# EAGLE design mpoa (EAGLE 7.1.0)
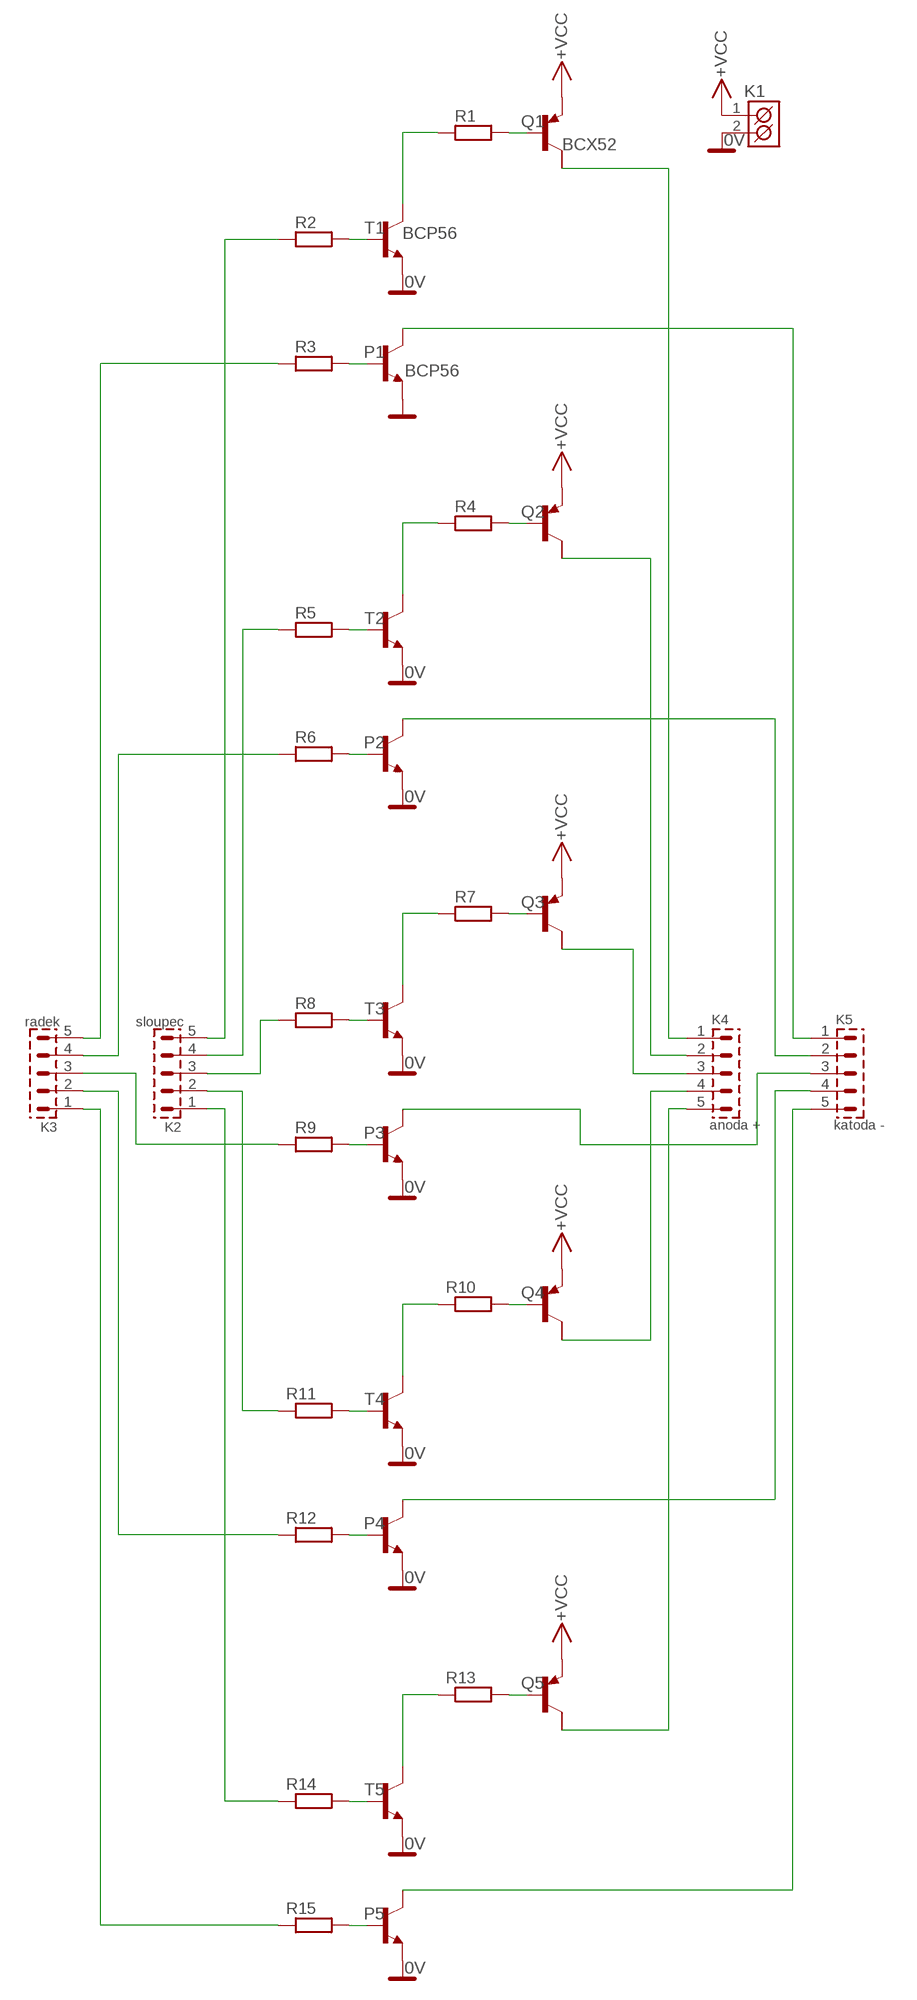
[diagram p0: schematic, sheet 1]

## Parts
K1  ARK550/2  [ARK550/2]
K2  sloupec  PSH02-05P  [PSH02-05P]
K3  radek  PSH02-05P  [PSH02-05P]
K4  anoda +  PSH02-05P  [PSH02-05P]
K5  katoda -  PSH02-05P  [PSH02-05P]
P1  -NPN-SOT223  [SOT223]
P2  -NPN-SOT223  [SOT223]
P3  -NPN-SOT223  [SOT223]
P4  -NPN-SOT223  [SOT223]
P5  -NPN-SOT223  [SOT223]
Q1  BCX52  PNP-TRANSISTIOR-2COLSOT89  [SOT89]
Q2  PNP-TRANSISTIOR-2COLSOT89  [SOT89]
Q3  PNP-TRANSISTIOR-2COLSOT89  [SOT89]
Q4  PNP-TRANSISTIOR-2COLSOT89  [SOT89]
Q5  PNP-TRANSISTIOR-2COLSOT89  [SOT89]
R1  R_1206  [1206]
R2  R_1206  [1206]
R3  R_1206  [1206]
R4  R_1206  [1206]
R5  R_1206  [1206]
R6  R_1206  [1206]
R7  R_1206  [1206]
R8  R_1206  [1206]
R9  R_1206  [1206]
R10  R_1206  [1206]
R11  R_1206  [1206]
R12  R_1206  [1206]
R13  R_1206  [1206]
R14  R_1206  [1206]
R15  R_1206  [1206]
T1  BCP56  -NPN-SOT223  [SOT223]
T2  -NPN-SOT223  [SOT223]
T3  -NPN-SOT223  [SOT223]
T4  -NPN-SOT223  [SOT223]
T5  -NPN-SOT223  [SOT223]

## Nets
0V: K1.2(K2) P1.3(E) P2.3(E) P3.3(E) P4.3(E) P5.3(E) T1.3(E) T2.3(E) T3.3(E) T4.3(E) T5.3(E) ; supply symbol labelled BCP56
N$1: K2.5 R2.1
N$2: R1.1 T1.4(C)
N$3: R2.2 T1.1(B)
N$4: Q1.1(B) R1.2
N$5: P1.1(B) R3.2
N$6: K2.3 R8.1
N$8: K4.1 Q1.2(C)
N$9: R5.2 T2.1(B)
N$10: Q2.1(B) R4.2
N$11: R4.1 T2.4(C)
N$12: P2.1(B) R6.2
N$13: K5.2 P2.4(C)
N$14: K4.2 Q2.2(C)
N$15: R8.2 T3.1(B)
N$16: Q3.1(B) R7.2
N$17: R7.1 T3.4(C)
N$18: P3.1(B) R9.2
N$19: K5.3 P3.4(C)
N$20: K4.3 Q3.2(C)
N$21: R11.2 T4.1(B)
N$22: Q4.1(B) R10.2
N$23: R10.1 T4.4(C)
N$24: P4.1(B) R12.2
N$25: K5.4 P4.4(C)
N$26: K4.4 Q4.2(C)
N$27: R14.2 T5.1(B)
N$28: Q5.1(B) R13.2
N$29: R13.1 T5.4(C)
N$30: P5.1(B) R15.2
N$32: K4.5 Q5.2(C)
N$34: K3.5 R3.1
N$35: K2.1 R14.1
N$36: K3.1 R15.1
N$37: K2.2 R11.1
N$38: K3.2 R12.1
N$39: K3.4 R6.1
N$40: K2.4 R5.1
N$41: K3.3 R9.1
N$42: K5.1 P1.4(C)
N$44: K5.5 P5.4(C)
VCC: K1.1(K1) Q1.3(E) Q2.3(E) Q3.3(E) Q4.3(E) Q5.3(E) ; supply symbol labelled +VCC
Unconnected: Q1.2@1(C/) Q2.2@1(C/) Q3.2@1(C/) Q4.2@1(C/) Q5.2@1(C/)

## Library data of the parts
K1 = #PaJa_konektory:ARK550/2: Svorkovnice - roztec 3,5mm - dvojita
K2-K5 = #PaJa_konektory:PSH02-05: Konektory se zamkem - vidlice - 5pin
P1-P5 T1-T5 = transistor-neu-to92:*-NPN-: NPN Transistror
Q1-Q5 = semicon-smd-ipc:PNP-TRANSISTIOR-2COL: PNP TRANSISTOR 2 colletor pins
R1-R15 = #PaJa_31:R: Rezistor

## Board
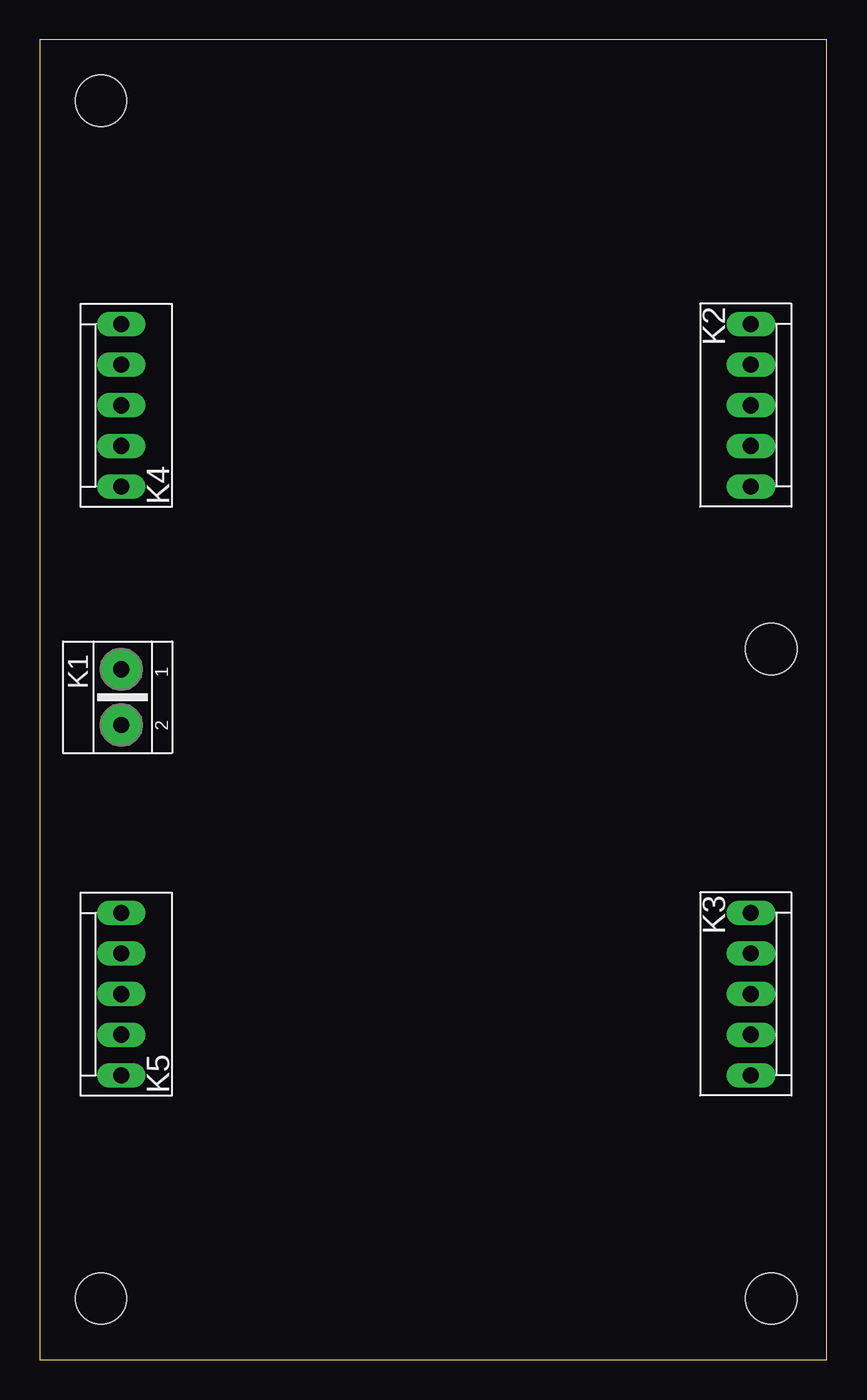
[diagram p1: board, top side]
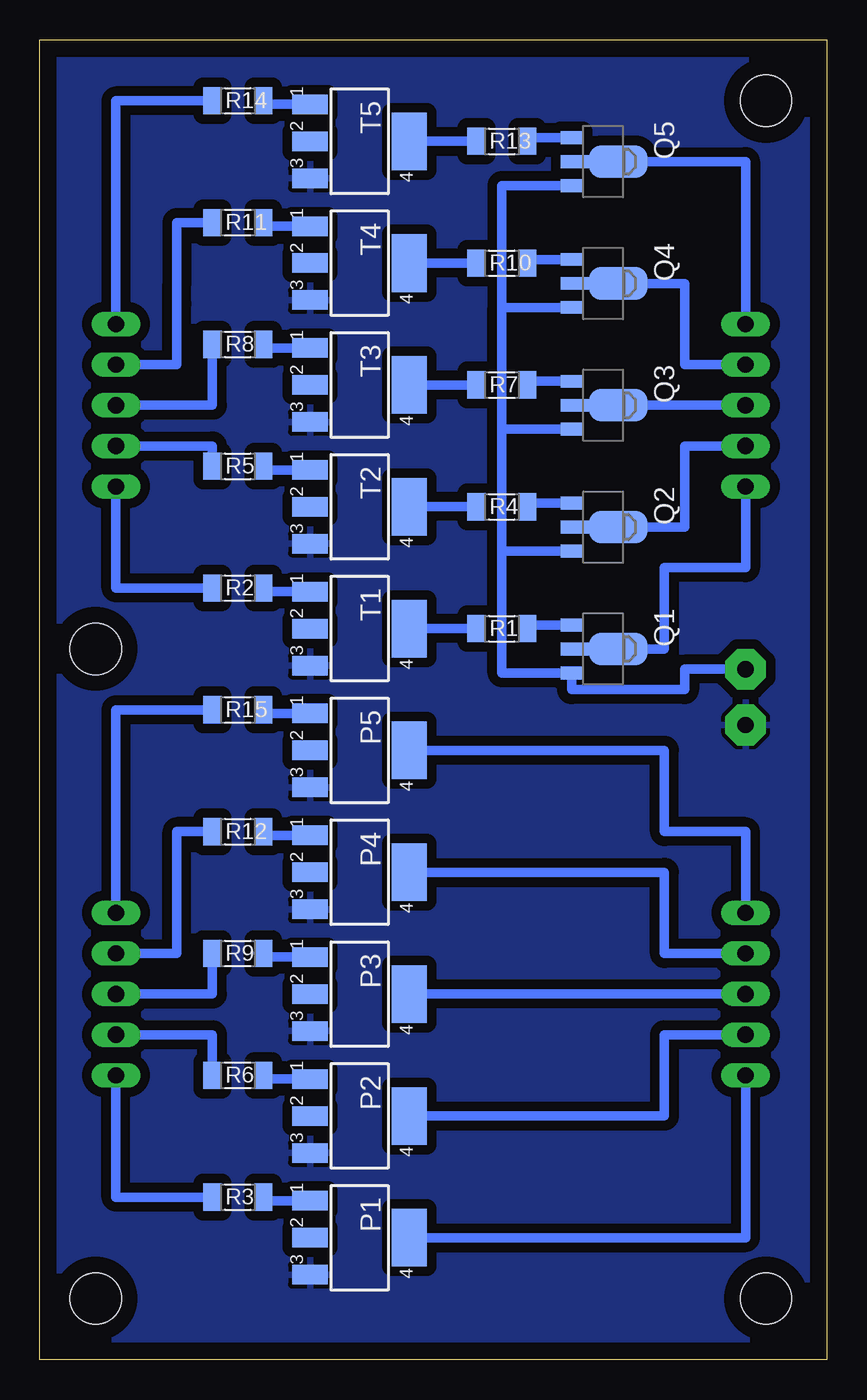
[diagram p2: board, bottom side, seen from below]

Size 49.2 x 82.54 mm. Coordinates in mm from the lower left corner, seen from the top.
Outline: 0,0 49.2,0 49.2,82.54 0,82.54 0,0
Copper layers (1*16): Top 0.035mm / dielectric 1.5mm / Bottom 0.035mm
Design rules "default": minimum track width 10mil, minimum drill 24mil, track to track 8mil, track to pad 8mil, pad to pad 8mil, via to via 8mil, smd to smd 8mil, copper to edge 40mil, drill to drill 8mil, minimum pad ring 10mil, minimum via ring 8mil, stop-mask expansion 4mil, vias tented up to drill 0mil, thermal gap 10mil
Holes 3.2 mm at 3.81,78.74 3.81,3.81 45.72,3.81 45.72,44.45

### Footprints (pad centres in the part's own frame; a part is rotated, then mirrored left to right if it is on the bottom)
ARK550/2 = drill 1.016 pad 2.54 octagon: 1 0,0; 2 3.493,0
PSH02-05P = drill 1.016 pad 1.422 long: 1 -5.08,0; 2 -2.54,0; 3 0,0; 4 2.54,0; 5 5.08,0
SOT223 = smd 1.219 x 2.235: 1 -2.311,-3.099; 2 0,-3.099; 3 2.311,-3.099 | smd 3.6 x 2.2: 4 0,3.099
SOT89 = smd 0.8 x 1.4: 1 -1.499,-1.981; 3 1.499,-1.981 | smd 0.8 x 1.9: 2 0,-1.727 | smd 2.032 x 3.65: 2@1 0,0.94
1206 = smd 1.143 x 1.702: 1 -1.587,0; 2 1.587,0

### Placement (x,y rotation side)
K1  5.08,43.18 270 top
K2  44.45,59.69 270 top
K3  44.45,22.86 270 top
K4  5.08,59.69 90 top
K5  5.08,22.86 90 top
P1  29.21,7.62 270 bottom
P2  29.21,15.24 270 bottom
P3  29.21,22.86 270 bottom
P4  29.21,30.48 270 bottom
P5  29.21,38.1 270 bottom
Q1  13.97,44.45 270 bottom
Q2  13.97,52.07 270 bottom
Q3  13.97,59.69 270 bottom
Q4  13.97,67.31 270 bottom
Q5  13.97,74.93 270 bottom
R1  20.32,45.72 0 bottom
R2  36.83,48.26 0 bottom
R3  36.83,10.16 0 bottom
R4  20.32,53.34 0 bottom
R5  36.83,55.88 0 bottom
R6  36.83,17.78 0 bottom
R7  20.32,60.96 0 bottom
R8  36.83,63.5 0 bottom
R9  36.83,25.4 0 bottom
R10  20.32,68.58 0 bottom
R11  36.83,71.12 0 bottom
R12  36.83,33.02 0 bottom
R13  20.32,76.2 0 bottom
R14  36.83,78.74 0 bottom
R15  36.83,40.64 0 bottom
T1  29.21,45.72 270 bottom
T2  29.21,53.34 270 bottom
T3  29.21,60.96 270 bottom
T4  29.21,68.58 270 bottom
T5  29.21,76.2 270 bottom

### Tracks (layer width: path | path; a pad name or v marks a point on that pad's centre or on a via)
0V
  pour Bottom (isolate 0.61): 1.27,81.28 48.26,81.28 48.26,1.27 1.27,1.27
N$1
  Bottom 0.61: R2.1 44.45,48.26 K2.5
N$2
  Bottom 0.61: R1.1 T1.4
N$3
  Bottom 0.61: T1.1 35.24,48.03 R2.2
N$4
  Bottom 0.61: Q1.1 18.73,45.95 R1.2
N$5
  Bottom 0.61: P1.1 35.24,9.93 R3.2
N$6
  Bottom 0.61: K2.3 38.42,59.69 R8.1
N$8
  Bottom 0.61: Q1.2 10.16,44.45 10.16,49.53 5.08,49.53 K4.1
N$9
  Bottom 0.61: T2.1 35.24,55.65 R5.2
N$10
  Bottom 0.61: Q2.1 18.73,53.57 R4.2
N$11
  Bottom 0.61: R4.1 T2.4
N$12
  Bottom 0.61: P2.1 35.24,17.55 R6.2
N$13
  Bottom 0.61: P2.4 10.16,15.24 10.16,20.32 K5.2
N$14
  Bottom 0.61: Q2.2 8.89,52.07 8.89,57.15 K4.2
N$15
  Bottom 0.61: T3.1 35.24,63.27 R8.2
N$16
  Bottom 0.61: Q3.1 18.73,61.19 R7.2
N$17
  Bottom 0.61: R7.1 T3.4
N$18
  Bottom 0.61: 35.56,25.4 R9.2 35.24,25.17 P3.1
N$19
  Bottom 0.61: K5.3 P3.4
N$20
  Bottom 0.61: K4.3 Q3.2
N$21
  Bottom 0.61: T4.1 35.24,70.89 R11.2
N$22
  Bottom 0.61: Q4.1 18.73,68.81 R10.2
N$23
  Bottom 0.61: R10.1 T4.4
N$24
  Bottom 0.61: P4.1 35.24,32.79 R12.2
N$25
  Bottom 0.61: P4.4 10.16,30.48 10.16,25.4 K5.4
N$26
  Bottom 0.61: Q4.2 8.89,67.31 8.89,62.23 K4.4
N$27
  Bottom 0.61: T5.1 35.24,78.51 R14.2
N$28
  Bottom 0.61: Q5.1 18.73,76.43 R13.2
N$29
  Bottom 0.61: T5.4 R13.1
N$30
  Bottom 0.61: P5.1 35.24,40.41 R15.2
N$32
  Bottom 0.61: Q5.2 5.08,74.93 K4.5
N$34
  Bottom 0.61: R3.1 44.45,10.16 K3.5
N$35
  Bottom 0.61: R14.1 44.45,78.74 K2.1
N$36
  Bottom 0.61: R15.1 44.45,40.64 K3.1
N$37
  Bottom 0.61: K2.2 40.64,62.23 40.64,66.04 40.64,67.31 40.64,71.12 R11.1
N$38
  Bottom 0.61: R12.1 40.64,33.02 40.64,25.4 K3.2
N$39
  Bottom 0.61: K3.4 38.42,20.32 R6.1
N$40
  Bottom 0.61: K2.4 38.42,57.15 R5.1
N$41
  Bottom 0.61: K3.3 38.42,22.86 R9.1
N$42
  Bottom 0.61: P1.4 5.08,7.62 K5.1
N$44
  Bottom 0.61: K5.5 5.08,33.02 10.16,33.02 10.16,38.1 P5.4
VCC
  Bottom 0.61: Q5.3 20.32,73.43 20.32,65.81 | Q4.3 20.32,65.81 | Q3.3 20.32,58.19 | 20.32,58.19 20.32,65.81 | Q2.3 20.32,50.57 | 20.32,50.57 20.32,58.19 | 20.32,50.57 20.32,42.95 Q1.3 15.95,41.91 8.89,41.91 8.89,43.18 K1.1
